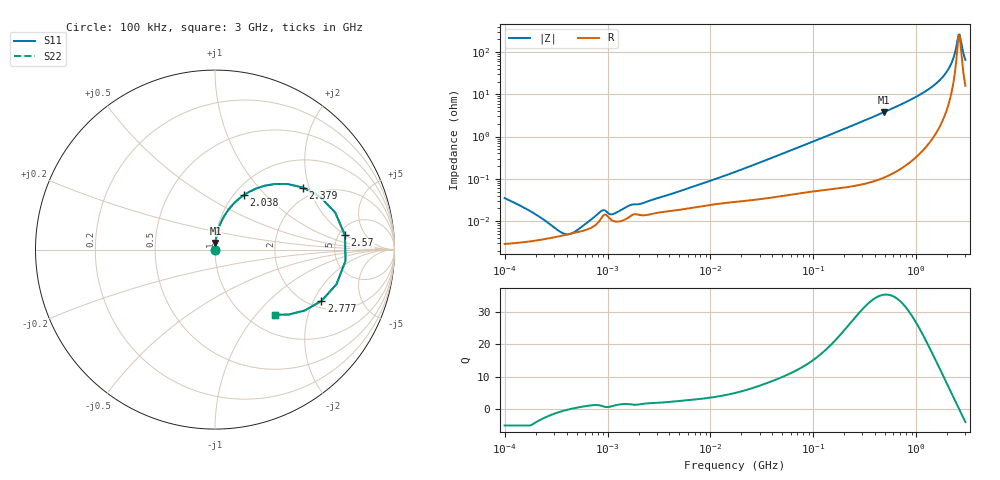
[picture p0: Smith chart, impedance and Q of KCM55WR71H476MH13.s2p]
!Murata Part Number: KCM55WR71H476MH13
!These Parameters are Measured in Series Mode Connection
!Data Generated on Mar 13, 2026
!  o--ll--o
!Port1  Port2
!  o------o
!Operation Temp=25[degC], DC Bias Voltage=0[V]
!Freq. Start=100[kHz] Stop=3[GHz] 401[Steps]
# Hz S RI R 50
!Freq.(Hz) S11(Real) S11(Imag) S21(Real) S21(Imag) S12(Real) S12(Imag) S22(Real) S22(Imag)
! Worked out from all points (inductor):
!   401 points, 100 kHz to 3 GHz, reference 50 ohm
!   read as one part in series: L = 1.41 nH near 7.028 MHz
!   highest Q = 35.4 at 481.3 MHz (marker M1), where L = 1.24 nH
!   self-resonance near 2.607 GHz
!   S11 on the Smith chart (normalised r, x): 100 kHz: 1.00, -0.00; 2.038 GHz: 1.11, +0.76; 2.379 GHz: 1.69, +1.83; 2.57 GHz: 5.68, +1.95; 2.777 GHz: 2.29, -2.31; 3 GHz: 1.32, -1.27
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100000  2.9e-05 -0.00035  1 0.00035  1 0.00035  2.9e-05 -0.00035
252895  3.81e-05 -9.12e-05  1 9.12e-05  1 9.12e-05  3.81e-05 -9.12e-05
562235  5.8e-05 4.52e-05  0.9999 -4.52e-05  0.9999 -4.52e-05  5.8e-05 4.52e-05
673391  6.72e-05 7.82e-05  0.9999 -7.82e-05  0.9999 -7.82e-05  6.72e-05 7.82e-05
894104  0.000129 0.000126  0.9999 -0.000126  0.9999 -0.000126  0.000129 0.000126
1127518  0.000102 0.000105  0.9999 -0.000105  0.9999 -0.000105  0.000102 0.000105
1659646  0.00013 0.0002  0.9999 -0.0002  0.9999 -0.0002  0.00013 0.0002
2092911  0.000139 0.000216  0.9999 -0.000216  0.9999 -0.000216  0.000139 0.000216
3161081  0.00016 0.00032  0.9998 -0.00032  0.9998 -0.00032  0.00016 0.00032
1.77727e7  0.000288 0.00146  0.9997 -0.00146  0.9997 -0.00146  0.000288 0.00146
9.738194e7  0.000555 0.00747  0.9994 -0.00747  0.9994 -0.00747  0.000555 0.00747
4.813181e8  0.00246 0.0373  0.9975 -0.0373  0.9975 -0.0373  0.00246 0.0373
5.475153e8  0.00306 0.0429  0.9969 -0.0429  0.9969 -0.0429  0.00306 0.0429
1.281618e9  0.0215 0.1226  0.9785 -0.1226  0.9785 -0.1226  0.0215 0.1226
1.746113e9  0.0686 0.2133  0.9314 -0.2133  0.9314 -0.2133  0.0686 0.2133
2.038117e9  0.1601 0.3032  0.8399 -0.3032  0.8399 -0.3032  0.1601 0.3032
2.201951e9  0.274 0.3552  0.726 -0.3552  0.726 -0.3552  0.274 0.3552
2.378954e9  0.4912 0.3454  0.5088 -0.3454  0.5088 -0.3454  0.4912 0.3454
2.570185e9  0.7241 0.0803  0.2759 -0.0803  0.2759 -0.0803  0.7241 0.0803
2.637286e9  0.727 -0.0631  0.273 0.0631  0.273 0.0631  0.727 -0.0631
2.776789e9  0.5928 -0.2864  0.4072 0.2864  0.4072 0.2864  0.5928 -0.2864
3e9  0.3357 -0.3631  0.6643 0.3631  0.6643 0.3631  0.3357 -0.3631
